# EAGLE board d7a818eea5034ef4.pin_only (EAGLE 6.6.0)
REV: B

Size 25.4 x 27.94 mm. Coordinates in mm from the lower left corner, seen from the top.
Outline: 2.54,0 22.86,0 arc90 25.4,2.54 25.4,25.4 arc90 22.86,27.94 2.54,27.94 arc90 0,25.4 0,2.54 arc90 2.54,0
Copper layers (1*16): Top 0.035mm / dielectric 1.5mm / Bottom 0.035mm
Design rules "adafruit *": minimum track width 8mil, minimum drill 15.5mil, track to track 8mil, track to pad 8mil, pad to pad 8mil, via to via 8mil, smd to smd 8mil, copper to edge 10mil, drill to drill 8mil, minimum pad ring 10mil, minimum via ring 8mil, stop-mask expansion 2mil, vias tented up to drill 20mil, thermal gap 10mil

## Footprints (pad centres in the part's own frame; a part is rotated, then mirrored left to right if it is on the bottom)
0805-NO = smd 1.24 x 1.5: 1 -0.95,0; 2 0.95,0
SOD-323 = smd 1.35 x 0.8: A 1.27,0; C -1.27,0
FIDUCIAL_1MM = smd 1 x 1: 1 0,0
1X08_ROUND_70 = drill 1 pad 1.778: 1 -8.89,0; 2 -6.35,0; 3 -3.81,0; 4 -1.27,0; 5 1.27,0; 6 3.81,0; 7 6.35,0; 8 8.89,0
SOLDERJUMPER_2WAY_OPEN_NOPASTE = smd 1.168 x 1.6: 1 -1.397,0; 2 0,0; 3 1.397,0
SOLDERJUMPER_ARROW_NOPASTE = smd 0.762 x 1.524: 1 -1.016,0; 2 1.016,0
QFN20_4MM_0.65MM = smd 0.35 x 0.95: 1 -1.3,-2.34; 2 -0.65,-2.34; 3 0,-2.34; 4 0.65,-2.34; 5 1.3,-2.34; 11 1.3,2.34; 12 0.65,2.34; 13 0,2.34; 14 -0.65,2.34; 15 -1.3,2.34 | smd 0.95 x 0.35: 6 2.34,-1.3; 7 2.34,-0.65; 8 2.34,0; 9 2.34,0.65; 10 2.34,1.3; 16 -2.34,1.3; 17 -2.34,0.65; 18 -2.34,0; 19 -2.34,-0.65; 20 -2.34,-1.3 | smd 3.25 x 3.25: PAD 0,0
SOT23-5 = smd 0.55 x 1.2: 1 -0.95,-1.3; 2 0,-1.3; 3 0.95,-1.3; 4 0.95,1.3; 5 -0.95,1.3
MOUNTINGHOLE_2.5_PLATED = drill 2.5 pad 3.2: P$1 0,0
TERMBLOCK_1X2-3.5MM = drill 1 pad 2.184: 1 1.8,0; 2 -1.7,0

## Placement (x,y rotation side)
C1  0.1uF  [0805-NO]  4.57,14.86 0 top
C2  0.1uF  [0805-NO]  17.27,9.78 0 top
C3  100nF  [0805-NO]  12.7,16.26 180 top
C4  10uF  [0805-NO]  4.57,5.97 0 top
C5  10uF  [0805-NO]  4.57,12.57 0 top
D1  1N4148  [SOD-323]  16.51,6.6 90 top
D2  1N4148  [SOD-323]  10.29,5.97 180 top
D3  1N4148  [SOD-323]  20.57,6.86 90 top
FB1  [0805-NO]  13.84,6.6 270 top
FID1  FIDUCIAL""  [FIDUCIAL_1MM]  23.75,21.72 90 top
FID2  FIDUCIAL""  [FIDUCIAL_1MM]  1.27,3.56 90 top
JP1  [1X08_ROUND_70]  12.7,2.67 0 top
R1  430Ω / 4300Ω 0.1%  [0805-NO]  17.53,11.94 180 top
R6  10K  [0805-NO]  18.54,6.6 270 top
R7  10K  [0805-NO]  22.61,6.86 270 top
R8  10K  [0805-NO]  7.24,6.73 270 top
SJ1  [SOLDERJUMPER_2WAY_OPEN_NOPASTE]  18.29,16 0 top
SJ3  [SOLDERJUMPER_ARROW_NOPASTE]  16.38,19.05 0 top
SJ4  [SOLDERJUMPER_ARROW_NOPASTE]  9.14,19.05 0 top
U1  MAX31865  [QFN20_4MM_0.65MM]  12.19,11.81 90 top
U3  MIC5225-3.3  [SOT23-5]  4.57,9.27 0 top
U$8  [PCBFEAT-REV-040]  1.4,7.87 0 top
U$16  [ADAFRUIT_3.5MM]  21.34,14.1 0 top
U$18  MOUNTINGHOLE2.5  [MOUNTINGHOLE_2.5_PLATED]  2.54,25.4 0 top
U$19  MOUNTINGHOLE2.5  [MOUNTINGHOLE_2.5_PLATED]  22.86,25.4 0 top
U$20  [ADAFRUIT_5MM]  5.71,18.29 0 bottom
U$21  [ADAFRUIT_5MM]  24.77,18.29 0 bottom
X1  3.5mm  [TERMBLOCK_1X2-3.5MM]  16.26,24.26 180 top
X2  3.5mm  [TERMBLOCK_1X2-3.5MM]  9.27,24.26 180 top

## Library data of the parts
C1-C5 D1-D3 FB1 JP1 R1 R6-R8 SJ1 U1 U3 U$8 U$16 U$20 U$21 X1 X2 = microbuilder
FID1 FID2 SJ3 SJ4 U$18 U$19 = microbuilder; BOM: EXCLUDE

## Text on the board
tPlace: F- | F+ | 2/3 Wire | RTD- | RTD+ | 2 Wire | MAX31865 | 24 | 3 | Rref | VIN | 3V3 | SDO | CS | GND | CLK | SDI | RDY
bPlace: F- | RTD- | RTD+ | F+ | MAX31865 | 2/3/4 Wire / Platinum RTD / Converter | Vin: 3-5VDC / Vlogic: 3-5VDC

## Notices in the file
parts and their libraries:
microbuilder: This work is placed in the public domain, and may be freely used for commercial and non-commercial work with the following conditions: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
